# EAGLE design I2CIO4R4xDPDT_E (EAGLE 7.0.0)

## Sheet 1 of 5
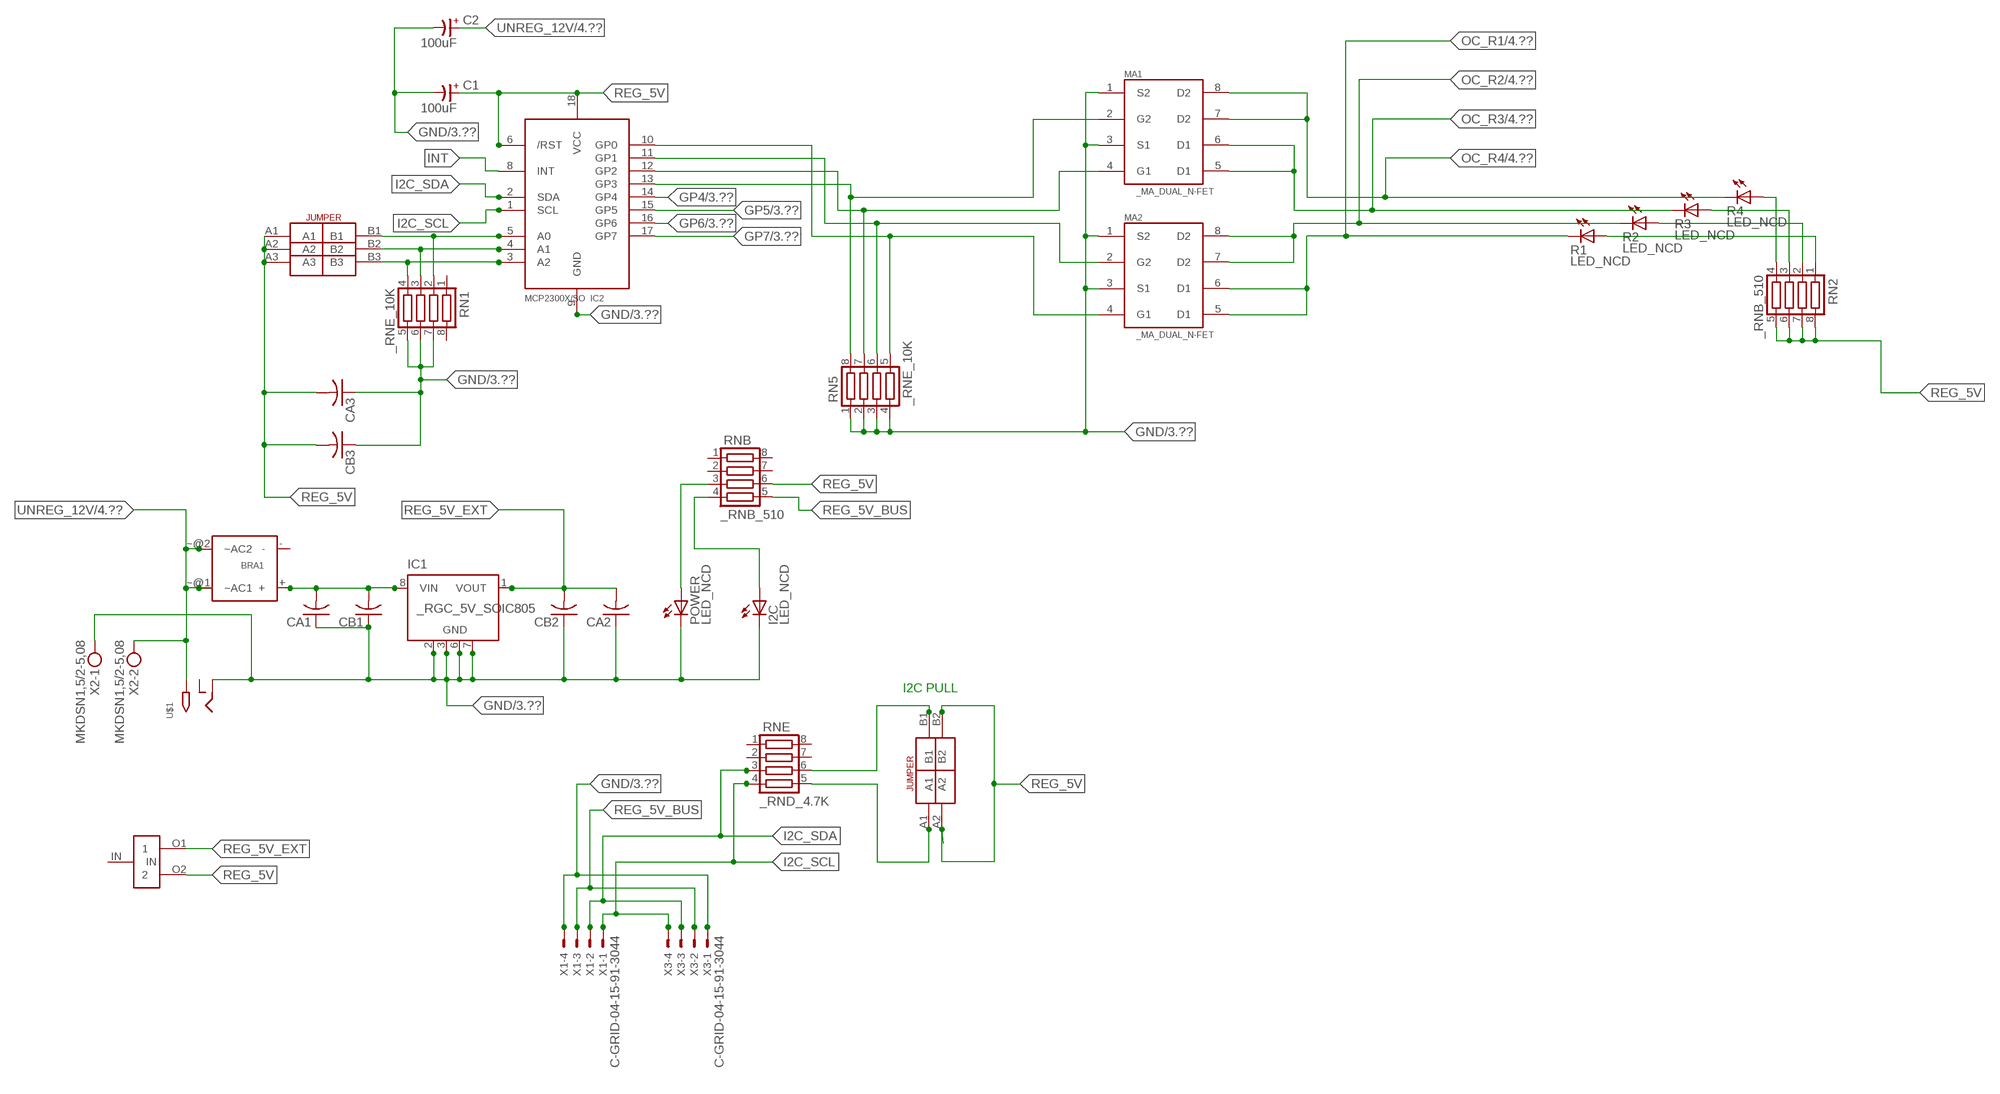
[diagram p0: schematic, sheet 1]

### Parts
BRA1  MB2S_  [MB2S]
C1  100uF  CP-E-025X060  [E-025X060]
C2  100uF  CP-E-025X060  [E-025X060]
CA1  CC1206KRX7R9BB104C1206K  [CC1206KRX7R9BB104]
CA2  CC1206KRX7R9BB104C1206K  [CC1206KRX7R9BB104]
CA3  CC1206KRX7R9BB104C1206K  [CC1206KRX7R9BB104]
CB1  TMK316F106ZL-TC1206K  [TMK316F106ZL-T]
CB2  TMK316F106ZL-TC1206K  [TMK316F106ZL-T]
CB3  TMK316F106ZL-TC1206K  [TMK316F106ZL-T]
I2C  LED_NCD  [CHIPLED_0603]
IC1  _RGC_5V_SOIC805  [_RGC_5V_SOIC8]
IC2  MCP2300X/SO  [SO18W]
MA1  _MA_DUAL_N-FET  [_MA_DUAL_N-FET]
MA2  _MA_DUAL_N-FET  [_MA_DUAL_N-FET]
POWER  LED_NCD  [CHIPLED_0603]
R1  LED_NCD  [CHIPLED_0603]
R2  LED_NCD  [CHIPLED_0603]
R3  LED_NCD  [CHIPLED_0603]
R4  LED_NCD  [CHIPLED_0603]
RN1  _RNE_10K  [RNE]
RN2  _RNB_510  [RNB]
RN5  _RNE_10K  [RNE]
RNB  _RNB_510  [RNB]
RNE  _RND_4.7K  [RND]
U$1  2.1MMJACK  [PJ-102A]
U$3  JUMPER_2X2  [JUMPER_2X2]
U$5  LINK_2  [LINK_2]
U$18  JUMPER_3X2  [JUMPER_3X2]
X1  C-GRID-04-15-91-3044  [15-91-04]
X2  MKDSN1,5/2-5,08  [MKDSN1,5/2-5,08]
X3  C-GRID-04-15-91-3044  [15-91-04]

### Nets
GND: C1.- C2.- CA1.1 CA2.1 CA3.1 CB1.1 CB2.1 CB3.1 I2C.C IC1.2(GND) IC1.3(GND) IC1.6(GND) IC1.7(GND) IC2.9(GND) MA1.1(S2) MA1.3(S1) MA2.1(S2) MA2.3(S1) POWER.C RN1.5 RN1.6 RN1.7 RN5.1 RN5.2 RN5.3 RN5.4 U$1.RING X1.4 X2.1 X3.1 ; also sheet 3
GP4: IC2.14(GP4) ; also sheet 3
GP5: IC2.15(GP5) ; also sheet 3
GP6: IC2.16(GP6) ; also sheet 3
GP7: IC2.17(GP7) ; also sheet 3
I2C_SCL: IC2.1(SCL) RNE.4 X1.1 X3.4
I2C_SDA: IC2.2(SDA) RNE.3 X1.2 X3.3
INT: IC2.8(INT)
N$1: BRA1.+ CA1.2 CB1.2 IC1.8(VIN)
N$2: POWER.A RNB.3
N$3: I2C.A RNB.4
N$4: RNE.5 U$3.A1
N$5: RNE.6 U$3.B1
N$6: IC2.5(A0) RN1.2 U$18.B1
N$7: IC2.4(A1) RN1.3 U$18.B2
N$8: IC2.3(A2) RN1.4 U$18.B3
N$20: IC2.13(GP3) MA1.2(G2) RN5.8
N$21: IC2.12(GP2) MA1.4(G1) RN5.7
N$22: IC2.11(GP1) MA2.2(G2) RN5.6
N$23: IC2.10(GP0) MA2.4(G1) RN5.5
N$29: R4.A RN2.4
N$30: R3.A RN2.3
N$31: R2.A RN2.2
N$32: R1.A RN2.1
OC_R1: MA2.5(D1) MA2.6(D1) R1.C ; also sheet 4
OC_R2: MA2.7(D2) MA2.8(D2) R2.C ; also sheet 4
OC_R3: MA1.5(D1) MA1.6(D1) R3.C ; also sheet 4
OC_R4: MA1.7(D2) MA1.8(D2) R4.C ; also sheet 4
REG_5V: C1.+ CA3.2 CB3.2 IC2.6(/RST) IC2.18(VCC) RN2.5 RN2.6 RN2.7 RN2.8 RNB.6 U$3.A2 U$3.B2 U$5.O2 U$18.A1 U$18.A2 U$18.A3
REG_5V_BUS: RNB.5 X1.3 X3.2
REG_5V_EXT: CA2.2 CB2.2 IC1.1(VOUT) U$5.O1
UNREG_12V: BRA1.~@1(~AC1) BRA1.~@2(~AC2) C2.+ U$1.TIP X2.2 ; also sheet 4
Unconnected: BRA1.- IC1.4(NC) IC1.5(NC) RN1.1 RN1.8 RNB.1 RNB.2 RNB.7 RNB.8 RNE.1 RNE.2 RNE.7 RNE.8 U$1.RING_SW U$5.IN

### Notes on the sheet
- I2C PULL

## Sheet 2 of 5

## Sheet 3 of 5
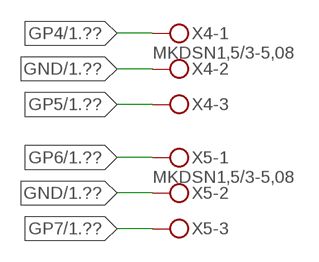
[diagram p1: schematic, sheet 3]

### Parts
X4  MKDSN1,5/3-5,08  [MKDSN1,5/3-5,08]
X5  MKDSN1,5/3-5,08  [MKDSN1,5/3-5,08]

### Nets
GND: X4.2 X5.2 ; also sheet 1
GP4: X4.1 ; also sheet 1
GP5: X4.3 ; also sheet 1
GP6: X5.1 ; also sheet 1
GP7: X5.3 ; also sheet 1

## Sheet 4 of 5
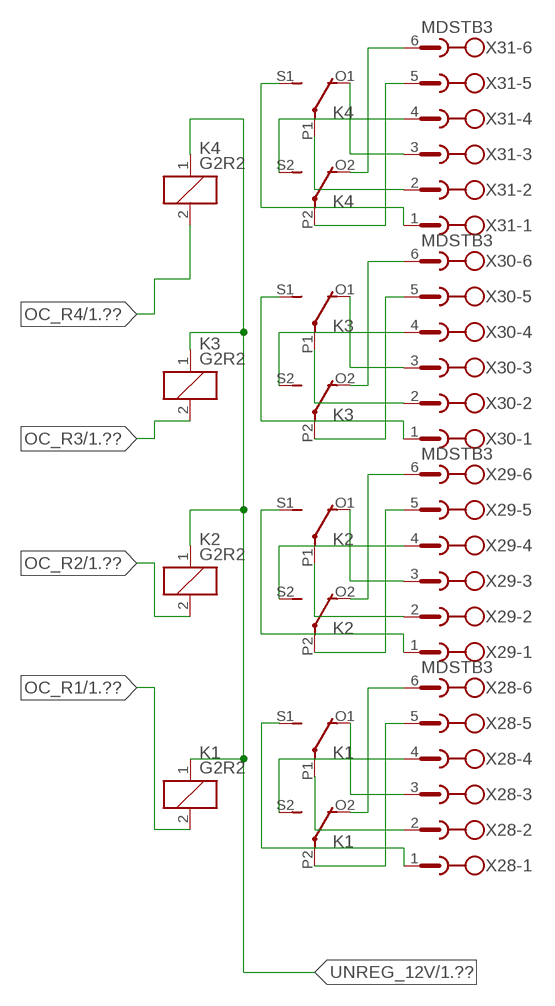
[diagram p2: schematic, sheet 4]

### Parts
K1  G2R2  [G2R2]
K2  G2R2  [G2R2]
K3  G2R2  [G2R2]
K4  G2R2  [G2R2]
X28  MDSTB3  [MDSTB3]
X29  MDSTB3  [MDSTB3]
X30  MDSTB3  [MDSTB3]
X31  MDSTB3  [MDSTB3]

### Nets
N$9: K3.P2(3:COM) X30.5
N$10: K3.O2(3:NC) X30.6
N$11: K4.P2(3:COM) X31.5
N$12: K4.O2(3:NC) X31.6
N$13: K3.S2(3:NO) X30.4
N$14: K4.S2(3:NO) X31.4
N$15: K3.O1(2:NC) X30.3
N$16: K4.O1(2:NC) X31.3
N$17: K4.P1(2:COM) X31.2
N$18: K3.P1(2:COM) X30.2
N$19: K3.S1(2:NO) X30.1
N$24: K4.S1(2:NO) X31.1
N$203: K1.P2(3:COM) X28.5
N$204: K1.O2(3:NC) X28.6
N$205: K1.S2(3:NO) X28.4
N$206: K1.P1(2:COM) X28.2
N$207: K1.O1(2:NC) X28.3
N$208: K1.S1(2:NO) X28.1
N$209: K2.P2(3:COM) X29.5
N$210: K2.O2(3:NC) X29.6
N$211: K2.S2(3:NO) X29.4
N$212: K2.S1(2:NO) X29.1
N$213: K2.P1(2:COM) X29.2
N$214: K2.O1(2:NC) X29.3
OC_R1: K1.2(1:C2) ; also sheet 1
OC_R2: K2.2(1:C2) ; also sheet 1
OC_R3: K3.2(1:C2) ; also sheet 1
OC_R4: K4.2(1:C2) ; also sheet 1
UNREG_12V: K1.1(1:C1) K2.1(1:C1) K3.1(1:C1) K4.1(1:C1) ; also sheet 1

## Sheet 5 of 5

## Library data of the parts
BRA1 = NCD_ULTIMATE_LIBRARY:MB2S: Bridge Rectifier BRA MB2S 200V 500ma Digikey MB2S-TPMSTR-ND/MB2S-TP
C1 C2 = NCD_ULTIMATE_LIBRARY:CP-: Capacitors All Kinds POLARIZED CAP
CA1-CA3 = NCD_ULTIMATE_LIBRARY:CC1206KRX7R9BB104: Capacitor CA .1uF 50V SMT C1206K CC1206KRX7R9BB104
CB1-CB3 = NCD_ULTIMATE_LIBRARY:TMK316F106ZL-T: Capacitor CB 10uF SMT 1206 TMK316F106ZL-T
I2C POWER = NCD_ULTIMATE_bhaskar:LED_NCD
IC1 = NCD_ULTIMATE_LIBRARY:_RGC_5V_SOIC8: Regulator Linear 5V Chip Positive VOLTAGE REGULATOR Digikey 497-7267-2-ND/L78L05CD13TR
IC2 = NCD_ULTIMATE_LIBRARY:MCP2300X: Semiconductor Port Expander I/O 8-Bit I2C MCP23008 Inexpensive i2c i/o expander - 8 general purpose i/o pins with optional pullups
K1-K4 = NCD_ULTIMATE_LIBRARY:G2R2: RELAY 2 x switch, Omron
MA1 MA2 = NCD_ULTIMATE_LIBRARY:_MA_DUAL_N-FET: FET Dual N-Channel 8-SOIC NMOSFET Digikey 785-1064-2-ND/AO4842
R1-R4 = NCD_ULTIMATE_LIBRARY:LED_NCD: LED Digikey 754-1132-2-ND/APT2012SRCPRV
RN1 RN5 = NCD_ULTIMATE_LIBRARY:_RNE_10K: Resistor Array RNE SMT 10K x 4 Single Resistor Source: http://www.ctscorp.com/components/Datasheets/CTSChipArrayDs.pdf Digikey 742C083103JPTR-ND/742C083103JP; OC_FARNELL: unknown; OC_NEWARK: unknown
RN2 RNB = NCD_ULTIMATE_LIBRARY:_RNB_510: Resistor Array RNB SMT 510 x 4 Single Resistor Source: http://www.ctscorp.com/components/Datasheets/CTSChipArrayDs.pdf Digikey 742C083511JPTR-ND/ 742C083511JP; OC_FARNELL: unknown; OC_NEWARK: unknown
RNE = NCD_ULTIMATE_LIBRARY:_RND_4.7K: Resistor Array RND SMT 4.7K x 4 Single Resistor Source: http://www.ctscorp.com/components/Datasheets/CTSChipArrayDs.pdf Digikey 742C083472JPTR-ND/742C083472JP; OC_FARNELL: unknown; OC_NEWARK: unknown
U$1 = NCD_ULTIMATE_CONNECTORS:2.1MMJACK: 2.1mm x 5.5mm DC jack with internal switch. Digikey part #PJ-102A, 4UCON part #05537 By microbuilder.eu
U$3 = NCD_ULTIMATE_CONNECTORS:JUMPER_2X2
U$5 = NCD_ULTIMATE_LIBRARY:LINK_2: PAD_top
U$18 = NCD_ULTIMATE_CONNECTORS:JUMPER_3X2
X1 X3 = NCD_ULTIMATE_CONNECTORS:C-GRID-04: CONNECTOR 4-Pos I2C wire to board 2.54 mm (0.100") pitch header Digikey WM1342-ND/0015912045; OC_FARNELL: unknown; OC_NEWARK: unknown
X2 = NCD_ULTIMATE_CONNECTORS:MKDSN1,5/2-5,08: MKDSN 1,5/ 2-5,08 Printklemme
X4 X5 = NCD_ULTIMATE_CONNECTORS:MKDSN1,5/3-5,08: MKDSN 1,5/ 3-5,08 Printklemme Nennstrom: 13,5 A Nennspannung: 250 V Rastermaß: 5,08 mm Polzahl: 3 Anschlussart: Schraubanschluss Montage: Löten Anschlussrichtung Leiter/Platine: 0 ° Artikelnummer: 1729131 Source: http://eshop.phoenixcontact.com .. 1729131.pdf
X28-X31 = NCD_ULTIMATE_LIBRARY:MDSTB3: PHOENIX

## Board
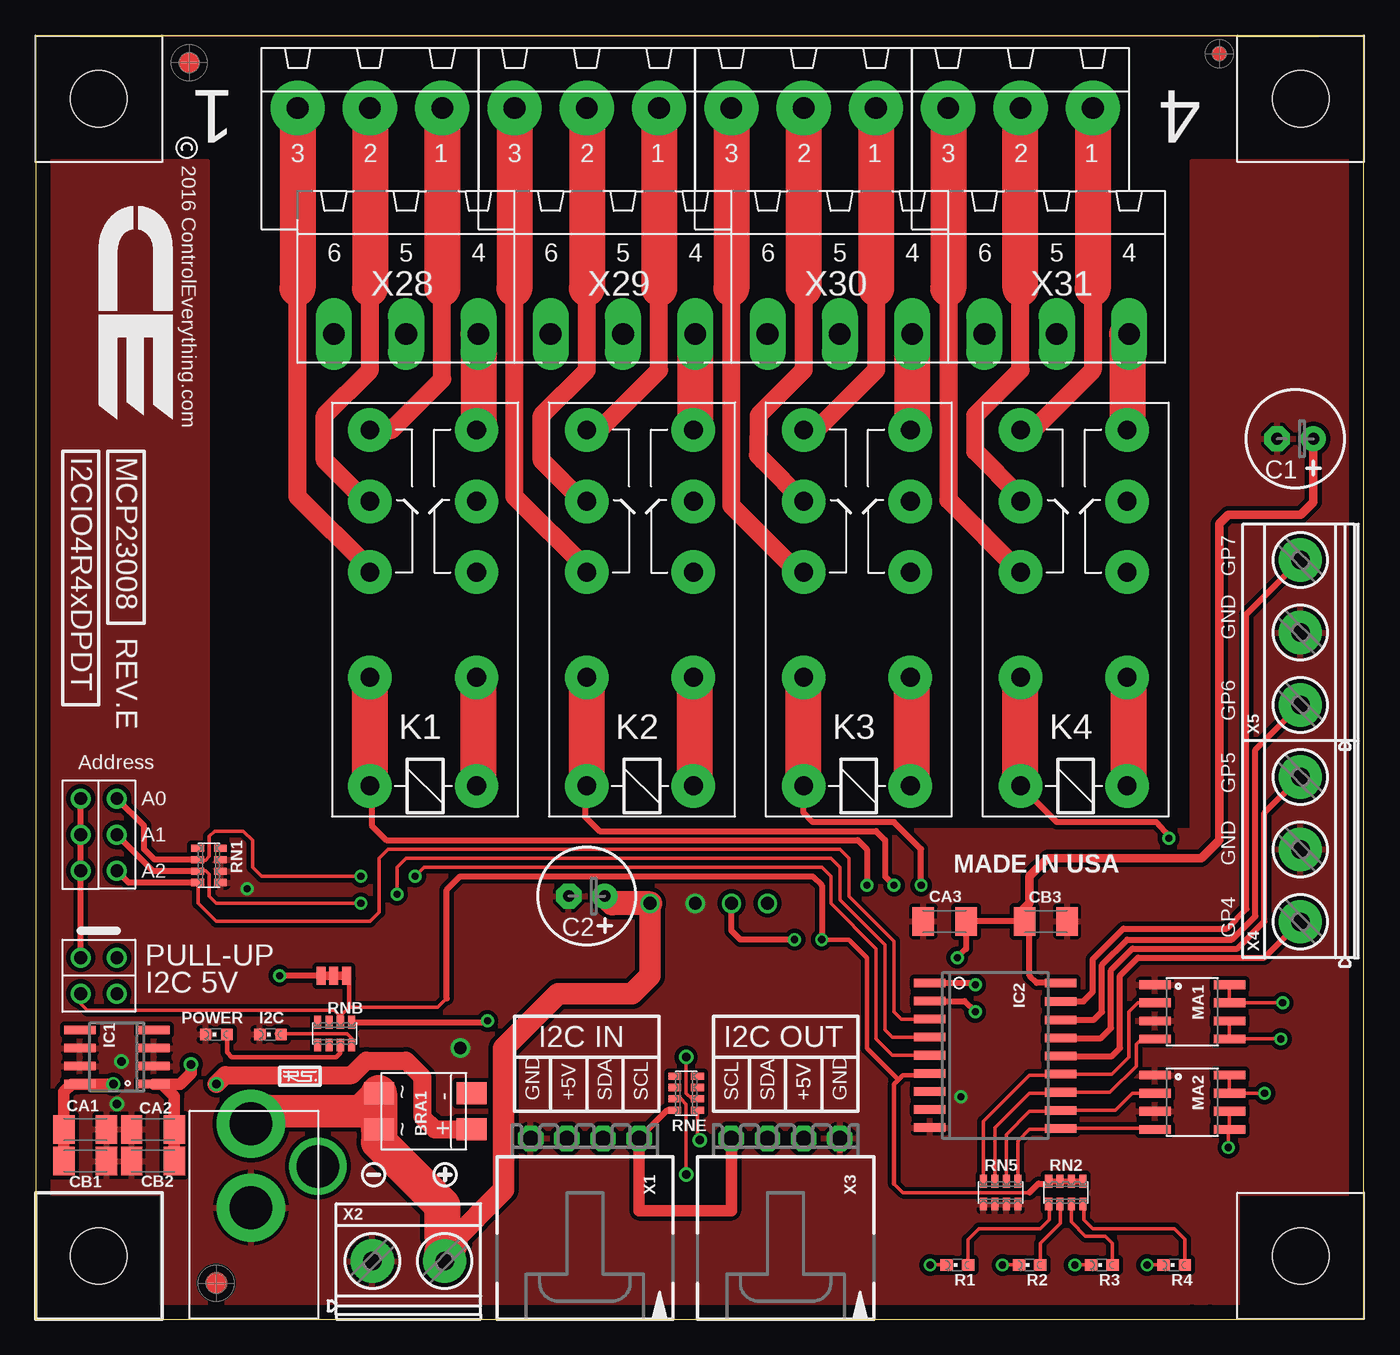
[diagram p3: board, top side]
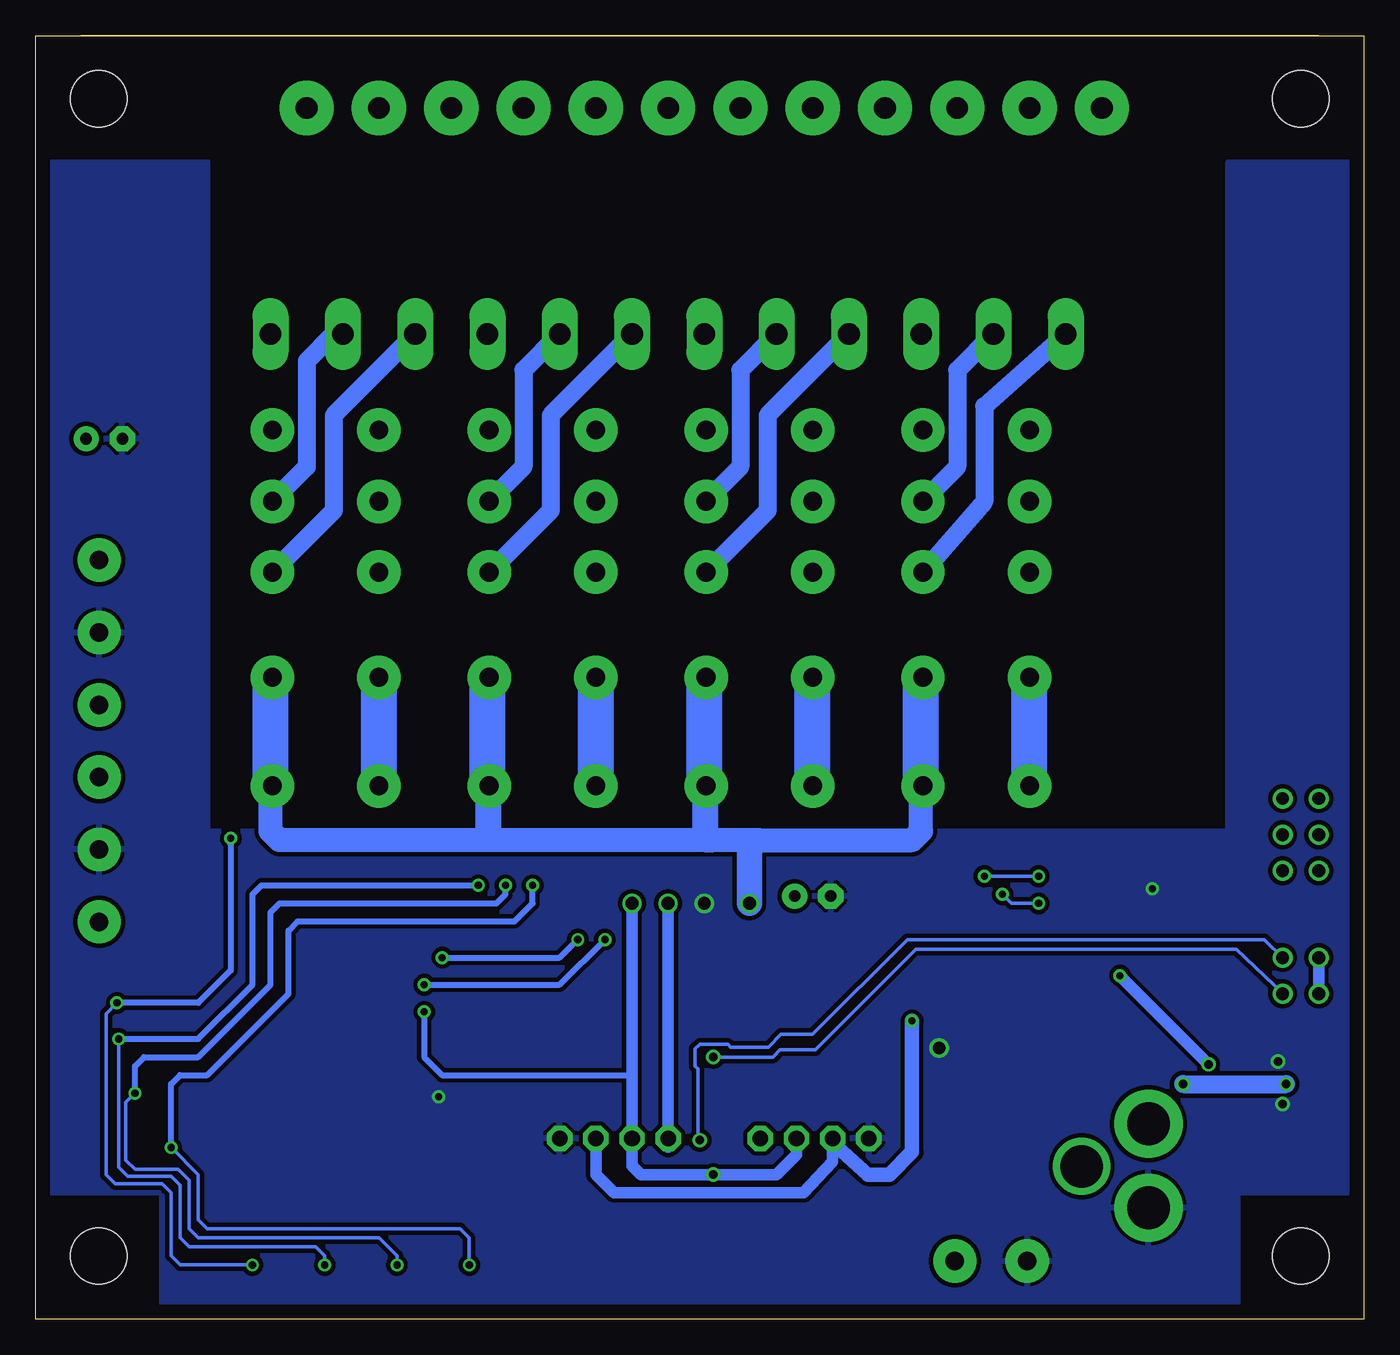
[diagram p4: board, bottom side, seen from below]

Size 93.34 x 90.17 mm. Coordinates in mm from the lower left corner, seen from the top.
Outline: 81.28,0 0,0 0,55.88
Outline: 81.28,0 82.53,0
Outline: 0,56.82 0,55.88
Outline: 81.28,0 93.34,0 93.34,90.17 0,90.17 0,55.88
Outline: 3.17,90.17 90.17,90.17
Copper layers (1*16): Top 0.035mm / dielectric 1.5mm / Bottom 0.035mm
Design rules "default": minimum track width 10mil, minimum drill 24mil, track to track 8mil, track to pad 8mil, pad to pad 8mil, via to via 8mil, smd to smd 8mil, copper to edge 40mil, drill to drill 8mil, minimum pad ring 10mil, minimum via ring 8mil, stop-mask expansion 4mil, vias tented up to drill 0mil, thermal gap 10mil
Holes 3.96 mm at 4.45,4.45

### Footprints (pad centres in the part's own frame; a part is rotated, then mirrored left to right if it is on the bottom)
MB2S = smd 1.55 x 2.1: + 0,-6.5; - 2.54,-6.5; ~@1 0,0; ~@2 2.54,0
E-025X060 = drill 0.813 pad 1.778: + -1.27,0 | drill 0.813 pad 1.778 octagon: - 1.27,0
CC1206KRX7R9BB104 = smd 1.5 x 2: 1 -1.5,0; 2 1.5,0
TMK316F106ZL-T = smd 1.5 x 2: 1 -1.5,0; 2 1.5,0
CHIPLED_0603 = smd 0.8 x 0.8: A 0,-0.75; C 0,0.75
_RGC_5V_SOIC8 = smd 0.6 x 2.2: 1 -1.905,-2.6; 2 -0.635,-2.6; 3 0.635,-2.6; 4 1.905,-2.6; 5 1.905,2.6; 6 0.635,2.6; 7 -0.635,2.6; 8 -1.905,2.6
SO18W = smd 0.6 x 2.2: 1 -4.445,-4.6; 2 -3.175,-4.6; 3 -1.905,-4.6; 4 -0.635,-4.6; 5 0.635,-4.6; 6 1.905,-4.6; 7 3.175,-4.6; 8 4.445,-4.6; 9 5.715,-4.6; 10 5.775,4.6; 11 4.505,4.6; 12 3.235,4.6; 13 1.965,4.6; 14 0.695,4.6; 15 -0.575,4.6; 16 -1.845,4.6; 17 -3.145,4.6; 18 -4.445,4.6
G2R2 = drill 1.321 pad 3.048: 1 -2.54,-3.683; 2 -2.54,3.81; 3 5.08,-3.683; 4 5.08,3.81; O1 12.471,3.81; O2 12.471,-3.683; P1 17.45,3.81; P2 17.45,-3.683; S1 22.454,3.81; S2 22.454,-3.683
_MA_DUAL_N-FET = smd 0.61 x 2.21: 1 -1.905,-2.616; 2 -0.635,-2.616; 3 0.635,-2.616; 4 1.905,-2.616; 5 1.905,2.616; 6 0.635,2.616; 7 -0.635,2.616; 8 -1.905,2.616
CHIPLED_0603' = smd 0.8 x 0.876: A 0,-0.75; C 0,0.75
RNE = smd 0.5 x 0.9: 1 -1.2,-0.8; 2 -0.4,-0.8; 3 0.4,-0.8; 4 1.2,-0.8; 5 1.2,0.8; 6 0.4,0.8; 7 -0.4,0.8; 8 -1.2,0.8
RNB = smd 0.5 x 0.9: 1 -1.2,-0.8; 2 -0.4,-0.8; 3 0.4,-0.8; 4 1.2,-0.8; 5 1.2,0.8; 6 0.4,0.8; 7 -0.4,0.8; 8 -1.2,0.8
RND = smd 0.5 x 0.9: 1 -1.2,-0.8; 2 -0.4,-0.8; 3 0.4,-0.8; 4 1.2,-0.8; 5 1.2,0.8; 6 0.4,0.8; 7 -0.4,0.8; 8 -1.2,0.8
PJ-102A = drill 3 pad 4.8: RING 0.1,-3.39; TIP 0.1,-9.29 | drill 3 pad 3.251: RING_SW -4.6,-6.29
JUMPER_2X2 = drill 0.9: A1 0,2.54; A2 0,0; B1 2.54,2.54; B2 2.54,0
PCB_MOUNTING_HOLE = hole 3.962: 4.445,4.445
LINK_2 = smd 1.27 x 0.635: IN 0,0; O1 0,0.889; O2 0,-0.889
JUMPER_3X2 = drill 0.9: A1 0,5.08; A2 0,2.54; A3 0,0; B1 2.54,5.08; B2 2.54,2.54; B3 2.54,0
15-91-04 = drill 1.1 pad 1.778 octagon: 1 -3.81,-7.62; 2 -1.27,-7.62; 3 1.27,-7.62; 4 3.81,-7.62
MKDSN1,5/2-5,08 = drill 1.3 pad 3.048: 1 -2.561,0.025; 2 2.519,0.025
MKDSN1,5/3-5,08 = drill 1.3 pad 3.048: 1 -7.641,0.025; 2 -2.561,0.025; 3 2.519,0.025
MDSTB3 = drill 1.524 pad 3.81: 1 -3.81,-10.795; 2 1.27,-10.795; 3 6.35,-10.795 | drill 1.524 pad 2.54 long: 4 -6.35,5.08; 5 -1.27,5.08; 6 3.81,5.08

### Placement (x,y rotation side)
BRA1  24.13,13.34 90 top
C1  88.52,61.85 180 top
C2  38.73,29.72 180 top
CA1  3.49,13.34 180 top
CA2  8.26,13.34 0 top
CA3  63.88,27.94 0 top
CB1  3.49,11.11 180 top
CB2  8.26,11.11 0 top
CB3  70.99,27.94 180 top
I2C  16.51,20 90 top
IC1  5.71,18.41 90 top
IC2  67.44,19.18 270 top
K1  27.3,40.01 90 top
K2  42.55,40.01 90 top
K3  57.78,40.01 90 top
K4  73.03,40.01 90 top
MA1  81.28,21.59 270 top
MA2  81.28,15.24 270 top
POWER  12.7,20 90 top
R1  LED_NCD  [CHIPLED_0603']  64.77,3.81 90 top
R2  LED_NCD  [CHIPLED_0603']  69.85,3.81 90 top
R3  LED_NCD  [CHIPLED_0603']  74.93,3.81 90 top
R4  LED_NCD  [CHIPLED_0603']  80.01,3.81 90 top
RN1  12.19,31.88 270 top
RN2  72.39,8.89 0 top
RN5  67.82,8.89 0 top
RNB  21.02,20.07 0 top
RNE  45.72,15.88 270 top
U$1  15.24,4.45 180 top
U$3  3.17,25.4 270 top
U$4  PCB_MOUNTING_HOLE  [PCB_MOUNTING_HOLE]  93.34,81.28 90 top
U$5  20.95,24.13 90 top
U$6  PCB_MOUNTING_HOLE  [PCB_MOUNTING_HOLE]  93.34,0 90 top
U$10  [VISION_REF15]  12.7,2.54 0 top
U$11  PCB_MOUNTING_HOLE  [PCB_MOUNTING_HOLE]  8.89,81.28 90 top
U$15  [VISION_REF15]  10.79,88.27 270 top
U$18  3.17,31.5 0 top
U$19  [VISION_REF10]  83.19,88.9 0 top
U$21  [ICON_USA]  64.52,31.37 0 top
U$22  [ICON_MINUS]  23.75,10.16 180 top
U$24  [ICON_PLUS]  28.77,10.16 90 top
X1  38.61,5.08 180 top
X2  26.23,4.06 0 top
X3  52.7,5.08 180 top
X4  88.9,35.56 90 top
X5  88.9,50.8 90 top
X28  24.77,74.3 180 top
X29  40.01,74.3 180 top
X30  55.24,74.3 180 top
X31  70.48,74.3 180 top

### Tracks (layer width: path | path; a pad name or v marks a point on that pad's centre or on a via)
GND  (via drill 0.5, 0.6, 0.9)
  Top 0.406: 34.8,12.38 X1.4
  Top 0.813: X3.1 56.52,12.06
  other vias: 5.71,15.11 6.03,18.1 46.35,29.21 29.84,19.05 14.86,30.23 65.02,15.62
  pour Bottom (isolate 0.305): 0.64,8.89 8.89,8.89 8.89,0 84.45,0 84.45,8.89 92.71,8.89 92.71,81.28 81.28,81.28 81.28,34.29 9.53,34.29 9.53,81.28 0.64,81.28
  pour Top (isolate 0.305): 0.64,8.89 8.89,8.89 8.89,0 84.45,0 84.45,8.89 92.71,8.89 92.71,81.28 81.28,81.28 81.28,34.29 12.06,34.29 12.06,81.28 0.64,81.28
GP4
  Top 0.406: IC2.14 75.63,18.48 76.2,19.05 76.2,24.13 77.47,25.4 86.36,25.4 X4.1
GP5
  Top 0.406: IC2.15 74.87,19.75 75.56,20.45 75.56,24.51 77.09,26.04 84.45,26.04 86.36,27.94 86.36,35.56 X4.3
GP6
  Top 0.406: IC2.16 74.36,21.02 74.93,21.59 74.93,24.89 76.71,26.67 84.07,26.67 85.72,28.32 85.72,40.01 X5.1
GP7
  Top 0.406: IC2.17 73.63,22.32 74.3,22.99 74.3,25.27 76.45,27.43 83.69,27.43 85.09,28.83 85.09,49.53 X5.3
I2C_SCL  (via drill 0.5, 0.9)
  Top 0.406: RNE.4 44.38,14.68 X1.1 | IC2.1 65.91,23.62 v66.04,23.5 | v53.34,26.67 49.53,26.67 48.9,27.3 v48.9,29.21
  Top 0.813: X3.4 48.9,7.62 42.42,7.62 X1.1
  Bottom 0.406: v66.04,23.5 56.52,23.5 v53.34,26.67
  Bottom 0.813: v48.9,29.21 X3.4 48.9,12.06
I2C_SDA  (via drill 0.5, 0.6, 0.9)
  Top 0.254: RNE.3 45.36,15.47 45.72,15.11 v45.72,10.16
  Top 0.406: IC2.2 65.28,22.35 v66.04,21.59
  Top 0.61: X3.3 51.44,12.06 | X1.2 39.88,12.38
  Bottom 0.406: v66.04,21.59 66.04,18.41 64.77,17.14 51.44,17.14 | 39.88,12.38 X1.2
  Bottom 0.813: 39.88,12.38 39.88,11.56 41.27,10.16 v45.72,10.16 50.8,10.16 51.44,10.79 X3.3 51.44,17.14 v51.44,29.21
N$1  (via drill 0.6)
  Top 0.813: CB1.2 CA1.2 1.99,15.96 2.54,16.51 IC1.8 v5.46,16.51
  Top 1.27: v12.7,16.51 13.34,17.14 22.23,17.14 23.24,18.16 26.04,18.16 27.18,17.02 27.18,14.22 28.07,13.34 BRA1.+
  Bottom 1.27: v12.7,16.51 v5.46,16.51
N$2
  Top 0.305: RNB.3 21.4,18.95 21.4,18.7 21.12,18.41 13.78,18.41 13.45,18.74 POWER.A
N$3
  Top 0.254: 22.23,18.95 22.23,19.74 21.9,20.07 16.94,20.07
  Top 0.305: RNB.4 22.23,18.95 | 16.94,20.07 I2C.A
N$4  (via drill 0.6)
  Top 0.254: RNE.5 46.52,12.6 v46.67,12.57
  Bottom 0.254: U$3.A1 6.99,26.67 32.07,26.67 38.73,20 40.96,20 41.85,19.11 44.51,19.11 44.7,19.3 46.67,19.3 46.99,18.99 46.99,17.78 46.8,17.59 46.8,12.7 v46.67,12.57
N$5  (via drill 0.6)
  Top 0.254: RNE.6 46.12,15.47 45.72,15.88 v45.72,18.41
  Bottom 0.254: v45.72,18.41 41.53,18.41 41.02,18.92 38.54,18.92 31.5,25.97 8.95,25.97 6.35,23.5 U$3.B1
N$6  (via drill 0.5)
  Top 0.254: IC2.5 60.2,18.54 59.05,19.68 59.05,26.04 55.88,29.21 55.88,31.11 55.24,31.75 27.3,31.75 v26.67,31.11 | v22.86,31.11 15.88,31.11 15.24,31.75 15.24,33.66 14.61,34.29 12.57,34.29 12.19,33.91 12.19,32.51 11.94,32.26 11.41,32.26 RN1.2
  Top 0.406: RN1.2 8.36,32.28 7.62,33.02 7.62,34.67 U$18.B1
  Bottom 0.254: v26.67,31.11 v22.86,31.11
N$7  (via drill 0.5)
  Top 0.254: IC2.4 60.2,19.81 59.69,20.32 59.69,26.29 56.52,29.46 56.52,31.75 55.88,32.38 26.04,32.38 25.4,31.75 v25.4,29.84 | v22.86,29.21 12.7,29.21 12.19,29.72 12.19,31.24 11.94,31.5 11.41,31.5 RN1.3
  Top 0.406: RN1.3 8.27,31.48 U$18.B2
  Bottom 0.254: v25.4,29.84 24.77,29.21 v22.86,29.21
N$8
  Top 0.254: IC2.3 60.83,21.08 60.33,21.59 60.33,26.54 57.15,29.72 57.15,32.38 56.52,33.02 24.77,33.02 24.13,32.38 24.13,28.57 23.5,27.94 12.7,27.94 11.43,29.21 11.43,30.64 RN1.4
  Top 0.406: RN1.4 6.53,30.68 U$18.B3
N$9
  Bottom 1.27: X30.5 59.05,66.67 59.05,59.87 K3.P2
N$10
  Bottom 1.27: X30.6 57.15,63.5 57.15,56.79 K3.O2
N$11
  Bottom 1.27: X31.5 72.39,69.22 74.3,67.31 74.3,59.87 K4.P2
N$12
  Bottom 1.27: X31.6 72.39,63.5 72.39,56.79 K4.O2
N$13
  Top 2.54: X30.4 61.59,62.59 K3.S2
N$14
  Top 2.54: X31.4 76.71,69.22 K4.S2
N$15
  Top 1.27: K3.O1 53.57,52.48 48.9,57.15 48.9,72.39
  Top 2.54: X30.3 48.9,72.39
N$16
  Top 1.27: 64.14,72.39 64.14,57.56 K4.O1
  Top 2.54: X31.3 64.14,72.39
N$17
  Top 1.27: K4.P1 69.22,57.78 66.04,60.96 66.04,63.5 69.22,66.67 69.22,72.39
  Top 2.54: 69.22,72.39 X31.2
N$18
  Top 1.27: 53.98,72.39 53.98,66.67 50.8,63.5 50.75,60.71 51.1,60.33 K3.P1
  Top 2.54: X30.2 53.98,72.39
N$19
  Top 1.27: 59.05,72.39 59.05,66.67 54.84,62.46 K3.S1
  Top 2.54: X30.1 59.05,72.39
N$20
  Top 0.254: MA1.2 77.47,22.23 76.83,21.59 76.83,18.41 75.63,17.21 IC2.13 71.97,17.14 69.85,17.14 66.62,13.91 RN5.8
N$21
  Top 0.254: MA1.4 77.72,19.68 77.34,19.3 77.34,17.78 75.5,15.94 IC2.12 71.97,15.88 69.85,15.88 67.42,13.44 RN5.7
N$22
  Top 0.254: MA2.2 77.09,15.88 75.89,14.67 IC2.11 71.97,14.61 69.85,14.61 68.22,12.97 RN5.6
N$23
  Top 0.254: MA2.4 78.6,13.4 IC2.10 71.97,13.34 69.85,13.34 69.02,12.5 RN5.5
N$24
  Top 1.27: 74.3,72.39 74.3,66.67 70.08,62.46 K4.S1
  Top 2.54: X31.1 74.3,72.39
N$29
  Top 0.254: R4.A 80.76,5.6 80.01,6.35 74.3,6.35 73.66,6.99 73.66,8.02 RN2.4
N$30
  Top 0.254: R3.A 75.68,5.35 75.18,5.84 73.79,5.84 72.77,6.86 72.77,8.07 RN2.3
N$31
  Top 0.254: R2.A 70.6,5.32 72.01,6.73 72.01,8.07 RN2.2
N$32
  Top 0.254: R1.A 65.52,5.58 66.29,6.35 70.61,6.35 71.25,6.99 71.25,8.03 RN2.1
N$203
  Bottom 1.27: X28.5 28.57,66.67 28.57,59.87 K1.P2
N$204
  Bottom 1.27: X28.6 26.67,64.14 26.67,57.43 K1.O2
N$205
  Top 2.54: X28.4 31.11,62.59 K1.S2
N$206
  Top 1.27: K1.P1 23.19,57.45 20.32,60.33 20.32,63.5 23.5,66.67 23.5,72.39
  Top 2.54: X28.2 23.5,72.39
N$207
  Top 1.27: K1.O1 23.5,52.7 18.41,57.78 18.41,72.39
  Top 2.54: X28.3 18.41,72.39
N$208
  Top 1.27: 28.57,72.39 28.57,66.04 24.99,62.46 K1.S1
  Top 2.54: X28.1 28.57,72.39
N$209
  Bottom 1.27: X29.5 43.81,66.67 43.81,59.87 K2.P2
N$210
  Bottom 1.27: X29.6 41.91,63.5 41.91,56.79 K2.O2
N$211
  Top 2.54: X29.4 46.35,62.59 K2.S2
N$212
  Top 1.27: 43.81,72.39 43.81,66.67 39.6,62.46 K2.S1
  Top 2.54: X29.1 43.81,72.39
N$213
  Top 1.27: K2.P1 38.43,57.45 35.56,60.33 35.56,63.5 38.73,66.67 38.73,72.39
  Top 2.54: X29.2 38.73,72.39
N$214
  Top 1.27: K2.O1 38.73,52.7 33.66,57.78 33.66,72.39
  Top 2.54: X29.3 33.66,72.39
OC_R1  (via drill 0.5)
  Top 0.254: R1.C v62.87,3.81 | v83.82,12.06 83.82,13.26 MA2.5 MA2.6
  Top 0.406: v58.42,30.48 58.42,33.02 57.78,33.66 24.64,33.66 23.62,34.67 23.62,37.21 23.5,37.21 K1.2
  Bottom 0.254: v62.87,3.81 62.87,5.71 63.5,6.35 81.28,6.35 81.92,6.99 81.92,10.16 v83.82,12.06
  Bottom 0.406: v83.82,12.06 83.82,16.51 83.19,17.14 81.28,17.14 75.56,22.86 75.56,27.3 74.93,27.94 59.69,27.94 58.42,29.21 v58.42,30.48
OC_R2  (via drill 0.5)
  Top 0.254: R2.C v67.94,3.81 | v86.36,15.88 MA2.7 MA2.8
  Top 0.406: v60.33,30.48 59.69,31.11 59.69,33.66 59.05,34.29 39.62,34.29 38.61,35.31 38.61,37.47 K2.2
  Bottom 0.254: v67.94,3.81 67.94,4.45 69.22,5.71 81.92,5.71 82.55,6.35 82.55,9.78 83.31,10.54 86.36,10.54 87,11.18 87,15.24 v86.36,15.88
  Bottom 0.406: v86.36,15.88 86.36,17.78 85.72,18.41 81.92,18.41 76.83,23.5 76.83,28.57 76.2,29.21 60.96,29.21 60.33,29.84 v60.33,30.48
OC_R3  (via drill 0.5)
  Top 0.254: R3.C v73.03,3.81 | v87.5,19.68 MA1.5 MA1.6
  Top 0.406: v62.23,30.48 62.23,33.02 60.33,34.92 54.61,34.92 53.98,35.56 K3.2
  Bottom 0.254: v73.03,3.81 73.03,4.45 73.66,5.08 82.55,5.08 83.19,5.71 83.19,9.4 83.82,10.03 86.87,10.03 87.5,10.67 v87.5,19.68
  Bottom 0.406: v87.5,19.68 81.92,19.68 78.11,23.5 78.11,29.84 77.47,30.48 v62.23,30.48
OC_R4  (via drill 0.5)
  Top 0.254: R4.C v78.11,3.81 | v87.63,22.23 MA1.7 MA1.8
  Top 0.406: v79.63,33.78 79.63,33.91 78.74,34.92 71.75,34.92 K4.2
  Bottom 0.254: v78.11,3.81 83.19,3.81 83.82,4.45 83.82,8.89 84.45,9.53 87.76,9.53 88.39,10.16 88.39,21.46 v87.63,22.23
  Bottom 0.406: v79.63,33.78 79.63,24.51 81.92,22.23 v87.63,22.23
REG_5V  (via drill 0.5)
  Top 0.229: 60.33,9.53 60.96,8.89 69.85,8.89
  Top 0.254: RNB.6 21.42,21.29 | 21.42,21.29 22.04,21.91 28.26,21.91 28.89,22.54 | 21.42,21.29 20.99,21.72 3.62,21.72 3.17,22.16 U$3.B2
  Top 0.305: 62.71,17.14 60.96,17.14 60.64,16.83 | 60.64,16.83 60.33,16.51 60.33,9.53 | 60.64,16.83 58.42,19.05 58.42,25.4 57.15,26.67 v55.24,26.67 | 22.04,21.91 22.04,23.94 U$5.O2
  Top 0.406: U$18.A1 U$18.A2 U$18.A3 U$3.A2 | IC2.18 70.36,23.62 69.85,24.13 69.85,27.58 CB3.2 CA3.2 65.38,26.01 v64.77,25.4 | 62.71,17.14 IC2.6 | 69.85,8.89 70.48,9.53 71.03,9.53 RN2.8 RN2.7 RN2.6 RN2.5 | 28.89,22.54 28.89,30.16 29.84,31.11 54.61,31.11 55.24,30.48 v55.24,26.67
  Top 0.61: C1.+ 89.79,57.4 88.9,56.52 83.82,56.52 83.19,55.88 83.19,33.66 81.92,32.38 71.12,32.38 69.85,31.11 69.85,29.21 69.22,28.57 69.22,28.22 CB3.2
  Bottom 0.406: v64.77,25.4 56.52,25.4 v55.24,26.67
  Bottom 0.813: U$3.B2 U$3.A2
REG_5V_BUS  (via drill 0.5)
  Top 0.406: RNB.5 31.66,20.87 v31.75,20.95
  Top 0.61: X1.3 37.34,12.38 | X3.2 53.98,12.06
  Bottom 0.406: 37.34,12.38 X1.3 | 53.98,12.06 X3.2
  Bottom 0.813: 37.34,12.38 37.34,11.05 39.37,8.89 52.7,8.89 53.98,10.16 53.98,12.06
  Bottom 1.016: 37.34,12.38 34.86,10.16 33.34,10.16 31.75,11.75 v31.75,20.95
REG_5V_EXT  (via drill 0.5, 0.6)
  Top 0.406: U$5.O1 v17.14,24.13
  Top 0.813: CB2.2 CA2.2 9.76,15.64 8.89,16.51 | 8.89,16.51 IC1.1 | v10.92,17.91 10.92,17.27 10.16,16.51 8.89,16.51
  Bottom 0.813: v17.14,24.13 v10.92,17.91
UNREG_12V  (via drill 0.9)
  Top 1.524: v43.18,29.21 43.18,24.13 41.91,22.86 36.7,22.86 32.89,19.05 32.89,9.08 29.11,5.3 28.57,4.76
  Top 1.676: v43.18,29.21 40.51,29.21 C2.+
  Top 2.286: BRA1.~@2 22.86,14.61 16.01,14.61
  Top 2.54: 16.01,14.61 U$1.TIP | X2.2 28.55,4.45 28.57,4.76 | BRA1.~@2 BRA1.~@1 24.13,12.45 28.57,8 28.57,5.84 29.11,5.3
  Bottom 1.676: 43.18,33.02 42.55,33.66 | 42.55,33.66 31.75,33.66 31.11,34.29 31.11,37.34 K1.1 | 42.55,33.66 45.72,33.66 | 45.72,33.66 46.35,34.29 46.35,37.34 K2.1 46.23,33.78 46.35,33.66 | 46.35,33.66 45.72,33.66 | 46.35,33.66 60.96,33.66 | 61.47,34.16 61.59,34.29 61.59,37.34 K3.1 61.47,34.16 | 61.47,34.16 60.96,33.66 | 60.96,33.66 76.2,33.66 76.83,34.29 76.83,37.34 K4.1
  Bottom 1.778: v43.18,29.21 43.18,33.02

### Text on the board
tNames: 1 | 4 | 2016 ControlEverything.com | I2CIO4R4xDPDT | MCP23008 | GP7 | REV.E | GND | GP6 | Address | GP5 | A0 | A1 | GND | A2 | GP4 | PULL-UP | I2C 5V | I2C IN | I2C OUT | GND | +5V | SDA | SCL | SCL | SDA | +5V | +5V | GND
